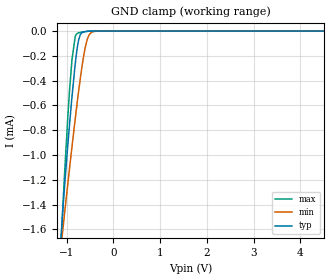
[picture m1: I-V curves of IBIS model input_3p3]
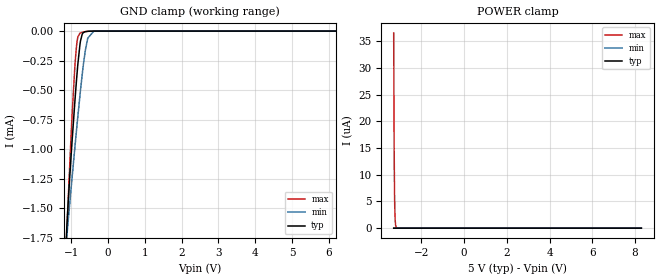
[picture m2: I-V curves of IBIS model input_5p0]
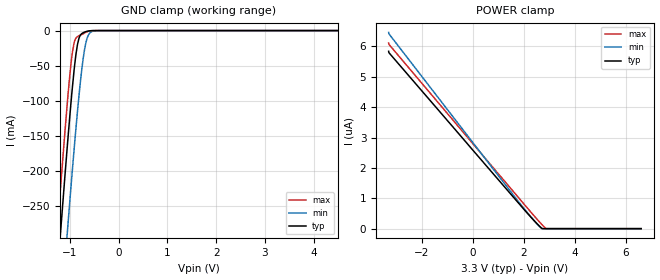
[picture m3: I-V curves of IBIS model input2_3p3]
|Texas Instruments Incorporated
| TIC12400-Q1 Automotive 24-Input Multiple Switch Detection Interface (MSDI)
| With Integrated ADC and Adjustable Wetting Current
| Marketing part#   Digital Voltage Range   Package-type   #pins
| TIC12400-Q1   3.0V-5.5V   TSSOP   38
[IBIS Ver]   4.1
[File name]   tic10024-q1.ibs
[Date]   08/08/2017
[File Rev]   1.0
[Source]
| Texas Instruments Incorporated.
| Analog-eLab Design Center, HPA
| 12500 TI Blvd
| Dallas, TX -75243
[Notes]
| Rev 1.0: 08/08/2017
| - Initial version of the model
| - Model generated from simulations in SPECTRE
| - Model matched to SPICE simulation
| - C_comp although listed in numerical order of value are
|   obtained from varying PVT conditions. For PVT conditions for
|   each specific value refer the buffer description under
|   respective [Model]. IBIS model user is responsible for using
|   appropriate C_comp to simulate for Signal Integrity.
| - Warnings regarding combined Non-monotonicity of various models
|   have been reviewed and considered minor and can be ignored.
[Disclaimer]
| This model is designed as an aid for customers of Texas Instruments.
| TI and its licensors and suppliers make no warranties, either expressed
| or implied, with respect to this  model, including the warranties of
| merchantability or fitness for a particular purpose. The model is
| provided solely on an "as is" basis. The entire risk as to its quality
| and performance is with the customer.
[Copyright]
(C) Copyright 2017 Texas Instruments Incorporated.All rights reserved.
|   TIC12400-Q1
[Component]   TIC12400-Q1
[Manufacturer]  TI
[Package]   |38 TSSOP - DCP package
|   typ   min   max
R_pkg   0.1   0.08   0.12
L_pkg   1.0nH   0.8nH   1.2nH
C_pkg   0.2pF   0.16pF   0.24pF
[Pin]  signal_name model_name   R_pin   L_pin   C_pin
1   IN13   nc   NA   NA   NA
2   IN14   nc   NA   NA   NA
3   IN15   nc   NA   NA   NA
4   IN16   nc   NA   NA   NA
5   IN17   nc   NA   NA   NA
6   IN18   nc   NA   NA   NA
7   IN19   nc   NA   NA   NA
8   IN20   nc   NA   NA   NA
9   AGND   gnd   NA   NA   NA
10   IN21   nc   NA   NA   NA
11   IN22   nc   NA   NA   NA
12   IN23   nc   NA   NA   NA
13   IN0   nc   NA   NA   NA
14   IN1   nc   NA   NA   NA
15   _CS   input   NA   NA   NA
16   SCLK   input   NA   NA   NA
17   SI   input   NA   NA   NA
18   SO   output   NA   NA   NA
19   VDD   power   NA   NA   NA
20   CAP_A   nc   NA   NA   NA
21   RESET   input2   NA   NA   NA
22   CAP_Pre   nc   NA   NA   NA
23   CAP_D   nc   NA   NA   NA
24   _INT   int   NA   NA   NA
25   IN2   nc   NA   NA   NA
26   IN3   nc   NA   NA   NA
27   IN4   nc   NA   NA   NA
28   DGND   gnd   NA   NA   NA
29   IN5   nc   NA   NA   NA
30   IN6   nc   NA   NA   NA
31   IN7   nc   NA   NA   NA
32   IN8   nc   NA   NA   NA
33   IN9   nc   NA   NA   NA
34   IN10   nc   NA   NA   NA
35   IN11   nc   NA   NA   NA
36   IN12   nc   NA   NA   NA
37   VS   power   NA   NA   NA
38   VS   power   NA   NA   NA
|   Model Selectors
[Model Selector] input
input_3p3   3.3V   digital Input
input_5p0   5.0V   digital Input
[Model Selector] input2
input2_3p3   3.3V   digital Input
input2_5p0   5.0V   digital Input
[Model Selector] int
int_3p3   3.3V  digital Output_open_drain
int_5p0   5.0V  digital Output_open_drain
[Model Selector] output
output_3p3   3.3V   digital Output
output_5p0   5.0V   digital Output
| Models and submodels in the file (8): input_3p3 (Input), input_5p0 (Input), input2_3p3 (Input), input2_5p0 (Input), int_3p3 (Open_drain), int_5p0 (Open_drain), output_3p3 (3-state), output_5p0 (3-state)
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|   input_3p3 Model
[Model]   input_3p3
Model_type   Input
Vinl = 0.99
Vinh = 2.31
|   typ   min   max
C_comp   2.62809E-14F   1.45091E-14F   2.8031E-14F
[Model spec]
|subparameter
Vinl   0.99   0.90   1.08
Vinh   2.31   2.10   2.52
| Where nom  PVT is Nominal Process, 3.3V, 27C
|   Fast PVT is Strong Process,  3.6V, -40C
|   Slow PVT is Weak Process,   3.0V, 150C
[Voltage Range]   3.3   3   3.6
|Junction Temperature
[Temperature Range]   27   150   -40
[Power Clamp Reference]   3.3   3   3.6
[GND Clamp Reference]   0   0   0
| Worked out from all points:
|   GND clamp passes 1 mA (typ) near -0.99 V on its own axis
[GND Clamp]
|   Voltage   I(typ)   I(min)   I(max)
-3.3V     -16.31mA   -13.01mA   -19.33mA
-1.181V   -2.029mA   -1.964mA   -2.18mA
-1.082V   -1.458mA   -1.61mA    -1.44mA
-973.5mV  -921uA     -1.234mA   -696.8uA
-884.4mV  -531.7uA   -934.6uA   -230.9uA
-815.1mV  -267.3uA   -710.2uA   -45.07uA
-755.7mV  -99.87uA   -526.7uA   -16.1uA
-696.3mV  -23.96uA   -356.4uA   -10.26uA
-567.6mV  -2.181uA   -80.97uA   -2.544uA
-488.4mV  -347.6nA   -17.29uA   -393.2nA
-399.3mV  -15.4nA    -2.342uA   -10.44nA
6.6V      0A         0A         0A
[POWER Clamp]
|   Voltage   I(typ)   I(min)   I(max)
-3.3V     0A         0A         0A
0V        0A         0A         0A
6.6V      0A         0A         0A
|   input_5p0 Model
[Model]   input_5p0
Model_type   Input
Vinl = 1.5
Vinh = 3.5
|   typ   min   max
C_comp   2.47536E-14F   1.61302E-14F   2.55646E-14F
[Model spec]
|subparameter
Vinl   1.5   1.35   1.65
Vinh   3.5   3.15   3.85
| Where nom  PVT is Nominal Process, 5.0V, 27C
|   Fast PVT is Strong Process,  5.5V, -40C
|   Slow PVT is Weak Process,   4.5V, 150C
[Voltage Range]   5   4.5   5.5
|Junction Temperature
[Temperature Range]   27   150   -40
[Power Clamp Reference]   5   4.5   5.5
[GND Clamp Reference]   0   0   0
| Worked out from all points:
|   GND clamp passes 1 mA (typ) near -0.99 V on its own axis
[GND Clamp]
|   Voltage   I(typ)   I(min)   I(max)
-3.3V     -16.31mA   -13.01mA   -19.33mA
-1.212V   -2.216mA   -2.078mA   -2.414mA
-1.108V   -1.597mA   -1.699mA   -1.625mA
-991.6mV  -1.005mA   -1.296mA   -811.1uA
-898.8mV  -591.8uA   -982.2uA   -293.1uA
-840.8mV  -359.4uA   -792.3uA   -88.86uA
-748mV    -84.6uA    -503.8uA   -15.01uA
-701.6mV  -27.33uA   -370.9uA   -10.65uA
-620.4mV  -5.27uA    -172uA     -5.265uA
-550.8mV  -1.578uA   -60.49uA   -1.871uA
-388.4mV  -8.43nA    -1.803uA   -4.384nA
8.3V      0A         0A         0A
[POWER Clamp]
|   Voltage   I(typ)   I(min)   I(max)
-3.3V     55.21pA    163.8pA    36.56uA
-3.288V   27.6pA     81.9pA     22.82uA
-3.277V   0A         0A         13.74uA
-3.265V   0A         0A         8.061uA
-3.254V   0A         0A         4.645uA
-3.242V   0A         0A         2.648uA
-3.23V    0A         0A         1.499uA
-3.219V   0A         0A         844.8nA
-3.196V   0A         0A         266.1nA
-3.161V   0A         0A         45.59nA
8.3V      0A         0A         0A
|   input2_3p3 Model
[Model]   input2_3p3
Model_type   Input
Vinl = 0.99
Vinh = 2.31
|   typ   min   max
C_comp   1.45761E-12F   1.38561E-12F   1.49155E-12F
[Model spec]
|subparameter
Vinl   0.99   0.90   1.08
Vinh   2.31   2.10   2.52
| Where nom  PVT is Nominal Process, 3.3V, 27C
|   Fast PVT is Strong Process,  3.6V, -40C
|   Slow PVT is Weak Process,   3.0V, 150C
[Voltage Range]   3.3   3   3.6
|Junction Temperature
[Temperature Range]   27   150   -40
[Power Clamp Reference]   3.3   3   3.6
[GND Clamp Reference]   0   0   0
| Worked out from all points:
|   GND clamp passes 1 mA (typ) near -0.65 V on its own axis
[GND Clamp]
|   Voltage   I(typ)   I(min)   I(max)
-3.3V     -2.326A    -2.432A    -2.273A
-1.27V    -360.5mA   -485.6mA   -296.5mA
-1.191V   -287.5mA   -412.6mA   -223.6mA
-1.053V   -164.5mA   -287.9mA   -102.8mA
-953.7mV  -84.5mA    -202.6mA   -33.43mA
-904.2mV  -50.27mA   -161.8mA   -15.07mA
-844.8mV  -20.03mA   -115.5mA   -8.552mA
-795.3mV  -7.818mA   -80.27mA   -6.746mA
-706.2mV  -2.39mA    -30.03mA   -3.774mA
-617.1mV  -561.7uA   -6.024mA   -944uA
-458.7mV  -7.002uA   -155.6uA   -7.387uA
6.6V      0A         0A         0A
[POWER Clamp]
|   Voltage   I(typ)   I(min)   I(max)
-3.3V     5.837uA    6.46uA     6.111uA
-3.29V    5.793uA    6.414uA    6.068uA
1.779V    855.4nA    901.8nA    1.036uA
2.383V    283.5nA    284.7nA    440.5nA
2.689V    23nA       15.64nA    153nA
2.888V    0A         0A         0A
6.6V      0A         0A         0A
